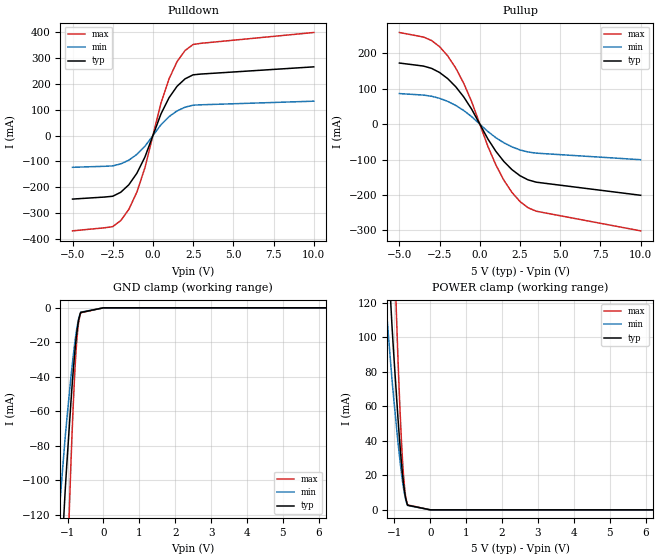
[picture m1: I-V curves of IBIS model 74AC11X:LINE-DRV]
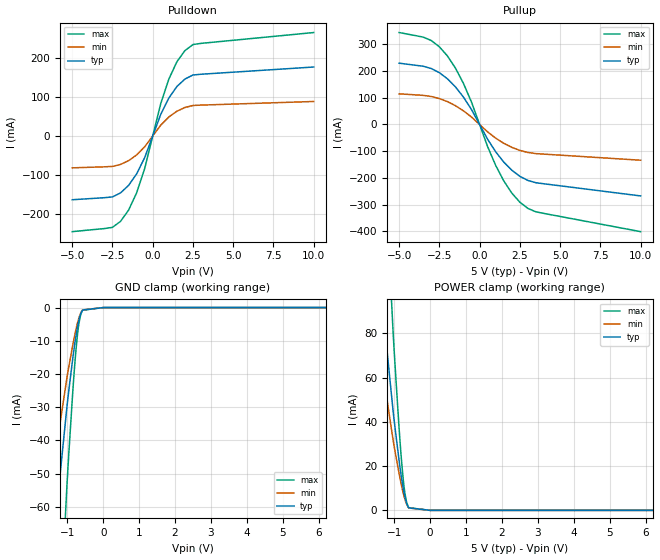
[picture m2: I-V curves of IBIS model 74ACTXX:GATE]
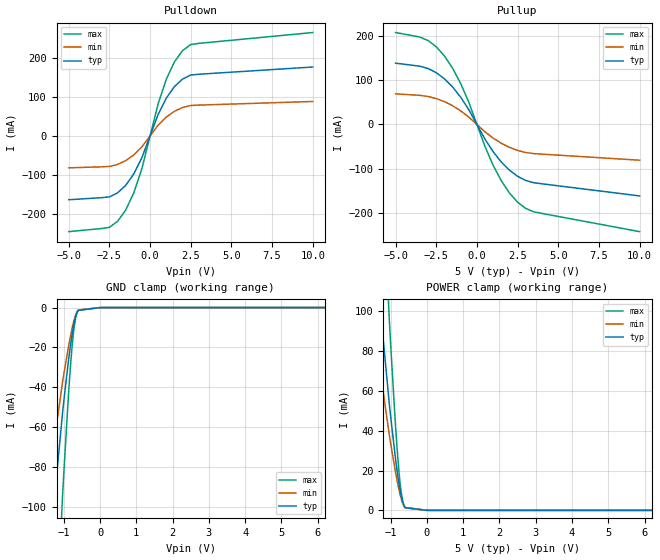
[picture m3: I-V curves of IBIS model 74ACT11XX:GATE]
|   This file is an IBIS representation of the   |
|   Mentor Graphics Corp.   |
|   generic   |
|=================== Header Section -------------------------------------------|
[IBIS Ver]   3.2
[File Name]   generic_mod.ibs
[File Rev]   0.1
[Date]   Mar 30, 2012
[Source]   This file originated at Mentor Graphics Corp.
   The original version of this file was automatically generated
   by the Easy IBIS Wizard v.4.1 (build 172)
[Notes]
   If you have comments concerning this file,
   please address them to:
   email: @
   phone:
[Disclaimer]   This information is for modeling purposes only, and is not
   guaranteed.
[Copyright]   Copyright (C)2012 Mentor Graphics Corp., All Rights Reserved
|------------------- End of Header Section ====================================|
|=================== Component Section ----------------------------------------|
[Component]   generic
[Manufacturer]  Mentor Graphics Corp.
[Package]
|   typ   min   max
R_pkg   10.000mOhm   5.000mOhm  15.000mOhm
L_pkg   2.000nH   1.000nH   3.000nH
C_pkg   0.800pF   0.400pF   1.200pF
[Pin] signal_name   model_name
1   74AC11X:LINE-DRV   74AC11X:LINE-DRV
2   74ACTXX:GATE   74ACTXX:GATE
3   74ACT11XX:GATE   74ACT11XX:GATE
4   74ACXX:LINE-DRV   74ACXX:LINE-DRV
5   74ACTXX:LINE-DRV   74ACTXX:LINE-DRV
6   74ACT11X:LINE-DRV   74ACT11X:LINE-DRV
7   74ALSXX:GATE   74ALSXX:GATE
8   74ALSXX:LINE-DRV   74ALSXX:LINE-DRV
9   74FCTXX:LINE-DRV   74FCTXX:LINE-DRV
10   74HCXX:GATE-2   74HCXX:GATE-2
11   74HCXX:OPEN-DRN   74HCXX:OPEN-DRN
12   74HCTXX:GATE-1   74HCTXX:GATE-1
13   74HCTXX:GATE-2   74HCTXX:GATE-2
14   74HCTXX:LINE-DRV   74HCTXX:LINE-DRV
15   74SXX:GATE   74SXX:GATE
16   16L8A:PLD   16L8A:PLD
17   26LS31   26LS31
18   DRAM_GENERIC   DRAM_GENERIC
19   TDR   TDR
20   74ACXX:GATE   74ACXX:GATE
21   74BCTXX:LINE-DRV   74BCTXX:LINE-DRV
22   74FXX:GATE   74FXX:GATE
23   74HCXX:GATE-1   74HCXX:GATE-1
24   74HCXX:LINE-DRV   74HCXX:LINE-DRV
25   74LSXX:GATE   74LSXX:GATE
26   74XX:OPEN-COL   74XX:OPEN-COL
27   BTL_(DS3896)   BTL_(DS3896)
28   DRAM,1Mx1   DRAM,1Mx1
29   LATTICE:16V8-10:PLD LATTICE:16V8-10:PLD
30   MACH:PLD   MACH:PLD
|------------------- End of Component Section =================================|
| Models and submodels in the file (30): 74AC11X:LINE-DRV (I/O), 74ACTXX:GATE (I/O), 74ACT11XX:GATE (I/O), 74ACXX:LINE-DRV (I/O), 74ACTXX:LINE-DRV (I/O), 74ACT11X:LINE-DRV (I/O), 74ALSXX:GATE (I/O), 74ALSXX:LINE-DRV (I/O), 74FCTXX:LINE-DRV (I/O), 74HCXX:GATE-2 (I/O), 74HCXX:OPEN-DRN (I/O_open_drain), 74HCTXX:GATE-1 (I/O), 74HCTXX:GATE-2 (I/O), 74HCTXX:LINE-DRV (I/O), 74SXX:GATE (I/O), 16L8A:PLD (I/O), 26LS31 (I/O), DRAM_GENERIC (I/O), TDR (I/O), 74ACXX:GATE (I/O), 74BCTXX:LINE-DRV (I/O), 74FXX:GATE (I/O), 74HCXX:GATE-1 (I/O), 74HCXX:LINE-DRV (I/O), 74LSXX:GATE (I/O), 74XX:OPEN-COL (I/O_open_drain), BTL_(DS3896) (I/O_open_drain), DRAM,1Mx1 (I/O), LATTICE:16V8-10:PLD (I/O), MACH:PLD (I/O)
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|=================== Models Section -------------------------------------------|
[Model]   74AC11X:LINE-DRV
Model_type   I/O
Polarity   Non-Inverting
Vinl  =   0.800V
Vinh  =   2.000V
Vmeas =   1.500V
Cref  =  50.000pF
Rref  =   1.000MOhm
Vref  =   0.000V
|   typ   min   max
C_comp   10.000pF   5.000pF   15.000pF
[Voltage Range]   5.000V   4.500V   5.500V
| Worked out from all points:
|   slope of the pulldown table from 0 to 0.75 V, typ, clamps not added: 6.55 ohm
|   slope of the pullup table from 0 to 0.75 V, typ, clamps not added: 12.7 ohm
[Pulldown]
| Voltage   I(typ)   I(min)   I(max)
-5V       -245.3mA   -122.6mA   -367.9mA
-2.5V     -234.3mA   -117.2mA   -351.5mA
-2V       -218.9mA   -109.4mA   -328.3mA
-1.5V     -190.1mA   -95.06mA   -285.2mA
-1V       -145.8mA   -72.88mA   -218.6mA
-500mV    -83.33mA   -41.67mA   -125mA
500mV     83.33mA    41.67mA    125mA
1V        145.8mA    72.88mA    218.6mA
1.5V      190.1mA    95.06mA    285.2mA
2V        218.9mA    109.4mA    328.3mA
3V        237.4mA    118.7mA    356.1mA
10V       265.1mA    132.6mA    397.7mA
[Pullup]
| Voltage   I(typ)   I(min)   I(max)
-5V       172.2mA    86.12mA    258.4mA
-3V       157.2mA    78.61mA    235.8mA
-2V       128.4mA    64.22mA    192.7mA
-1.5V     105.6mA    52.79mA    158.4mA
-1V       76.76mA    38.38mA    115.1mA
-500mV    41.67mA    20.83mA    62.5mA
500mV     -41.67mA   -20.83mA   -62.5mA
1V        -76.76mA   -38.38mA   -115.1mA
1.5V      -105.6mA   -52.79mA   -158.4mA
2.5V      -145.6mA   -72.78mA   -218.3mA
3.5V      -163.6mA   -81.82mA   -245.5mA
10V       -200.7mA   -100.3mA   -301mA
[GND Clamp]
| Voltage   I(typ)   I(min)   I(max)
-5V       -1.627A    -1.09A     -3.228A
-1.069V   -106.5mA   -75.37mA   -190.7mA
-1.017V   -89.04mA   -63.62mA   -156.6mA
-907.7mV  -54.62mA   -40.28mA   -90.16mA
-855.5mV  -39.76mA   -30.06mA   -62.37mA
-808.2mV  -27.74mA   -21.64mA   -40.79mA
-768.6mV  -19.05mA   -15.4mA    -26.1mA
-749.3mV  -15.39mA   -12.7mA    -20.27mA
-692.5mV  -7.18mA    -6.349mA   -8.397mA
-634.6mV  -2.693mA   -2.54mA    -2.876mA
0V        0A         0A         0A
10V       0A         0A         0A
[POWER Clamp]
| Voltage   I(typ)   I(min)   I(max)
-5V       1.627A     1.09A      3.228A
-1.069V   106.5mA    75.37mA    190.7mA
-1.017V   89.04mA    63.62mA    156.6mA
-907.7mV  54.62mA    40.28mA    90.16mA
-855.5mV  39.76mA    30.06mA    62.37mA
-808.2mV  27.74mA    21.64mA    40.79mA
-768.6mV  19.05mA    15.4mA     26.1mA
-749.3mV  15.39mA    12.7mA     20.27mA
-692.5mV  7.18mA     6.349mA    8.397mA
-634.6mV  2.693mA    2.54mA     2.876mA
0V        0A         0A         0A
10V       0A         0A         0A
[Ramp]
|   typ   min   max
dV/dt_r   2.375V/1.440ns   1.699V/2.592ns   2.820V/1.056ns
dV/dt_f   2.672V/1.140ns   2.121V/2.052ns   3.056V/836.000ps
R_load =  50.000Ohm
|------------------- End of 74AC11X:LINE-DRV ----------------------------------
[Model]   74ACTXX:GATE
Model_type   I/O
Polarity   Non-Inverting
Vinl  =   0.800V
Vinh  =   2.000V
Vmeas =   1.500V
Cref  =  50.000pF
Rref  =   1.000kOhm
Vref  =   0.000V
|   typ   min   max
C_comp   5.000pF   2.500pF   7.500pF
[Voltage Range]   5.000V   4.500V   5.500V
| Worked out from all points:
|   slope of the pulldown table from 0 to 0.75 V, typ, clamps not added: 9.82 ohm
|   slope of the pullup table from 0 to 0.75 V, typ, clamps not added: 9.5 ohm
|   GND clamp passes 1 mA (typ) near -0.59 V on its own axis
[Pulldown]
| Voltage   I(typ)   I(min)   I(max)
-5V       -163.5mA   -81.76mA   -245.3mA
-2.5V     -156.2mA   -78.11mA   -234.3mA
-2V       -145.9mA   -72.97mA   -218.9mA
-1.5V     -126.8mA   -63.38mA   -190.1mA
-1V       -97.17mA   -48.58mA   -145.8mA
-500mV    -55.56mA   -27.78mA   -83.33mA
500mV     55.56mA    27.78mA    83.33mA
1V        97.17mA    48.58mA    145.8mA
1.5V      126.8mA    63.38mA    190.1mA
2V        145.9mA    72.97mA    218.9mA
3V        158.2mA    79.12mA    237.4mA
10V       176.8mA    88.38mA    265.1mA
[Pullup]
| Voltage   I(typ)   I(min)   I(max)
-5V       229.7mA    114.8mA    344.5mA
-3V       209.6mA    104.8mA    314.4mA
-2V       171.3mA    85.63mA    256.9mA
-1.5V     140.8mA    70.39mA    211.2mA
-1V       102.3mA    51.17mA    153.5mA
-500mV    55.56mA    27.78mA    83.33mA
500mV     -55.56mA   -27.78mA   -83.33mA
1V        -102.3mA   -51.17mA   -153.5mA
1.5V      -140.8mA   -70.39mA   -211.2mA
2.5V      -194.1mA   -97.04mA   -291.1mA
3.5V      -218.2mA   -109.1mA   -327.3mA
10V       -267.6mA   -133.8mA   -401.4mA
[GND Clamp]
| Voltage   I(typ)   I(min)   I(max)
-5V       -458.6mA   -307.2mA   -910mA
-1.008V   -29.6mA    -20.95mA   -53.03mA
-956.2mV  -24.75mA   -17.69mA   -43.53mA
-846.8mV  -15.18mA   -11.19mA   -25.05mA
-794.5mV  -11.05mA   -8.352mA   -17.33mA
-747.3mV  -7.706mA   -6.013mA   -11.33mA
-707.6mV  -5.291mA   -4.277mA   -7.25mA
-650.8mV  -2.646mA   -2.283mA   -3.218mA
-625.9mV  -1.829mA   -1.629mA   -2.116mA
-573.6mV  -748.1uA   -705.5uA   -799uA
0V        0A         0A         0A
10V       0A         0A         0A
[POWER Clamp]
| Voltage   I(typ)   I(min)   I(max)
-5V       684.7mA    458.6mA    1.359A
-1.028V   44.39mA    31.42mA    79.52mA
-975.5mV  37.12mA    26.52mA    65.28mA
-866.1mV  22.76mA    16.79mA    37.57mA
-813.8mV  16.57mA    12.53mA    26mA
-766.6mV  11.56mA    9.019mA    17mA
-726.9mV  7.936mA    6.416mA    10.87mA
-670.1mV  3.968mA    3.425mA    4.827mA
-645.2mV  2.744mA    2.443mA    3.175mA
-592.9mV  1.122mA    1.058mA    1.198mA
0V        0A         0A         0A
10V       0A         0A         0A
[Ramp]
|   typ   min   max
dV/dt_r   2.518V/1.200ns   1.907V/2.160ns   2.938V/880.000ps
dV/dt_f   2.500V/1.200ns   1.841V/2.160ns   2.931V/880.000ps
R_load =  50.000Ohm
|------------------- End of 74ACTXX:GATE --------------------------------------
[Model]   74ACT11XX:GATE
Model_type   I/O
Polarity   Non-Inverting
Vinl  =   0.800V
Vinh  =   2.000V
Vmeas =   1.500V
Cref  =  50.000pF
Rref  =   1.000kOhm
Vref  =   0.000V
|   typ   min   max
C_comp   5.000pF   2.500pF   7.500pF
[Voltage Range]   5.000V   4.500V   5.500V
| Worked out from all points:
|   slope of the pulldown table from 0 to 0.75 V, typ, clamps not added: 9.82 ohm
|   slope of the pullup table from 0 to 0.75 V, typ, clamps not added: 15.8 ohm
[Pulldown]
| Voltage   I(typ)   I(min)   I(max)
-5V       -163.5mA   -81.76mA   -245.3mA
-2.5V     -156.2mA   -78.11mA   -234.3mA
-2V       -145.9mA   -72.97mA   -218.9mA
-1.5V     -126.8mA   -63.38mA   -190.1mA
-1V       -97.17mA   -48.58mA   -145.8mA
-500mV    -55.56mA   -27.78mA   -83.33mA
500mV     55.56mA    27.78mA    83.33mA
1V        97.17mA    48.58mA    145.8mA
1.5V      126.8mA    63.38mA    190.1mA
2V        145.9mA    72.97mA    218.9mA
3V        158.2mA    79.12mA    237.4mA
10V       176.8mA    88.38mA    265.1mA
[Pullup]
| Voltage   I(typ)   I(min)   I(max)
-5V       137.8mA    68.9mA     206.7mA
-3V       125.8mA    62.89mA    188.7mA
-2V       102.8mA    51.38mA    154.1mA
-1.5V     84.46mA    42.23mA    126.7mA
-1V       61.41mA    30.7mA     92.11mA
-500mV    33.33mA    16.67mA    50mA
500mV     -33.33mA   -16.67mA   -50mA
1V        -61.41mA   -30.7mA    -92.11mA
1.5V      -84.46mA   -42.23mA   -126.7mA
2.5V      -116.5mA   -58.23mA   -174.7mA
3.5V      -130.9mA   -65.46mA   -196.4mA
10V       -160.6mA   -80.28mA   -240.8mA
[GND Clamp]
| Voltage   I(typ)   I(min)   I(max)
-5V       -820mA     -549.2mA   -1.627A
-1.036V   -53.26mA   -37.7mA    -95.41mA
-984.1mV  -44.54mA   -31.82mA   -78.32mA
-874.8mV  -27.32mA   -20.14mA   -45.09mA
-822.5mV  -19.88mA   -15.03mA   -31.19mA
-775.2mV  -13.87mA   -10.82mA   -20.4mA
-735.6mV  -9.524mA   -7.699mA   -13.05mA
-678.8mV  -4.762mA   -4.11mA    -5.792mA
-653.9mV  -3.293mA   -2.932mA   -3.809mA
-601.6mV  -1.347mA   -1.27mA    -1.438mA
0V        0A         0A         0A
10V       0A         0A         0A
[POWER Clamp]
| Voltage   I(typ)   I(min)   I(max)
-5V       820mA      549.2mA    1.627A
-1.036V   53.26mA    37.7mA     95.41mA
-984.1mV  44.54mA    31.82mA    78.32mA
-874.8mV  27.32mA    20.14mA    45.09mA
-822.5mV  19.88mA    15.03mA    31.19mA
-775.2mV  13.87mA    10.82mA    20.4mA
-735.6mV  9.524mA    7.699mA    13.05mA
-678.8mV  4.762mA    4.11mA     5.792mA
-653.9mV  3.293mA    2.932mA    3.809mA
-601.6mV  1.347mA    1.27mA     1.438mA
0V        0A         0A         0A
10V       0A         0A         0A
[Ramp]
|   typ   min   max
dV/dt_r   2.231V/1.500ns   1.522V/2.700ns   2.712V/1.100ns
dV/dt_f   2.500V/1.200ns   1.841V/2.160ns   2.931V/880.000ps
R_load =  50.000Ohm
|------------------- End of 74ACT11XX:GATE ------------------------------------
